PROGRAM AMCI_Motion_Sample
VAR
	
FB_relative_move_1: relative_move_dut; 
b_relative_move_1_en: BOOL;
b_relative_move_1_er: BOOL; 

FB_absolute_move_1: absolute_move_dut; 
b_absolute_move_1_en: BOOL;
b_absolute_move_1_er: BOOL; 

FB_jog_CW_1: jog_cw_dut; 
b_jog_cw_1_en: BOOL;
b_jog_cw_1_er: BOOL; 

FB_jog_CCW_1: jog_ccw_dut; 
b_jog_ccw_1_en: BOOL;
b_jog_ccw_1_er: BOOL; 

FB_home_cw_1: home_cw_dut; 
b_home_cw_1_en: BOOL;
b_home_cw_1_er: BOOL; 

FB_reset_errors_1: reset_errors_dut;  

FB_Preset_1: preset_dut;  
b_preset_1_en: BOOL;
b_preset_1_er: BOOL; 

FB_hold_1: hold_dut;  
b_hold_1_en: BOOL;
b_hold_1_er: BOOL; 

b_comment_coil_1: bool; 

END_VAR
VAR // added by the converter: edge detectors and wires of the graphical bodies
    _w1, _w2, _w3, _w4, _w5, _w6, _w7 : BOOL;
END_VAR

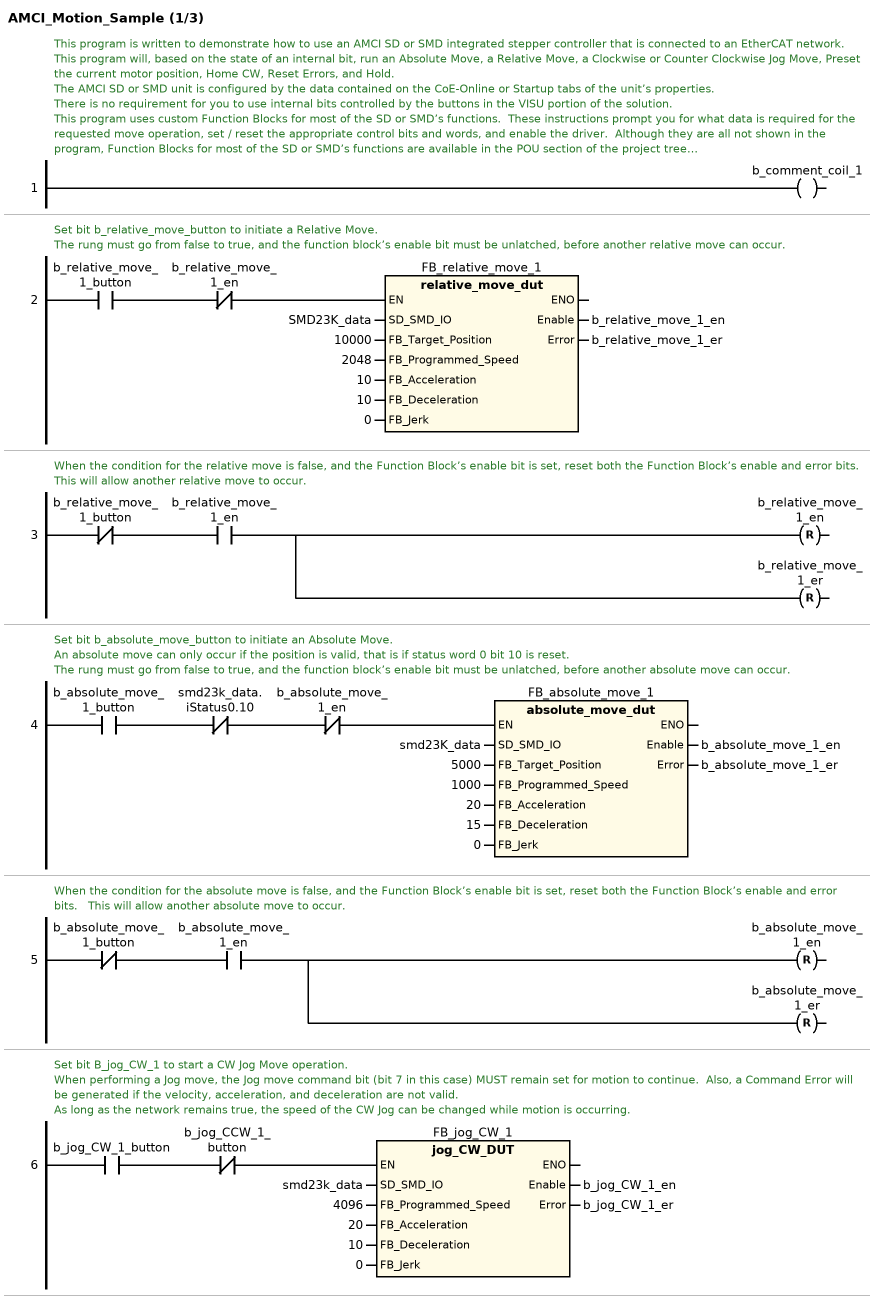
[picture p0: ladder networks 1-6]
// NETWORK 1
// This program is written to demonstrate how to use an AMCI SD or SMD integrated stepper controller that is connected to an EtherCAT network.  This program will, based on the state of an internal bit, run an Absolute Move, a Relative Move, a Clockwise or Counter Clockwise Jog Move, Preset the current motor position, Home CW, Reset Errors, and Hold.
//
// The AMCI SD or SMD unit is configured by the data contained on the CoE-Online or Startup tabs of the unit’s properties.
//
// There is no requirement for you to use internal bits controlled by the buttons in the VISU portion of the solution.
//
// This program uses custom Function Blocks for most of the SD or SMD’s functions.  These instructions prompt you for what data is required for the requested move operation, set / reset the appropriate control bits and words, and enable the driver.  Although they are all not shown in the program, Function Blocks for most of the SD or SMD’s functions are available in the POU section of the project tree.
//
// The custom Function Blocks will only function if a variable with the AMCI_DUT_STEPPER Data Unit Type was linked to the input and output data from the SD or SMD unit.
//
// This program will work correctly only if one button / function is true at a time.
//
// This sample program has a routine containing a Function Block for programming and running Assembled Moves.  Ignore or delete this routine if you are not using this function.
b_comment_coil_1 := TRUE;

// NETWORK 2
// Set bit b_relative_move_button to initiate a Relative Move.
//
// The rung must go from false to true, and the function block’s enable bit must be unlatched, before another relative move can occur.
IF b_relative_move_1_button AND NOT b_relative_move_1_en THEN
    FB_relative_move_1(
        SD_SMD_IO := SMD23K_data,
        FB_Target_Position := 10000,
        FB_Programmed_Speed := 2048,
        FB_Acceleration := 10,
        FB_Deceleration := 10,
        FB_Jerk := 0,
        Enable => b_relative_move_1_en,
        Error => b_relative_move_1_er); // relative_move_dut
END_IF

// NETWORK 3
// When the condition for the relative move is false, and the Function Block’s enable bit is set, reset both the Function Block’s enable and error bits.   This will allow another relative move to occur.
_w1 := NOT b_relative_move_1_button AND b_relative_move_1_en;
b_relative_move_1_en R= _w1;
b_relative_move_1_er R= _w1;

// NETWORK 4
// Set bit b_absolute_move_button to initiate an Absolute Move.
//
// An absolute move can only occur if the position is valid, that is if status word 0 bit 10 is reset.
//
// The rung must go from false to true, and the function block’s enable bit must be unlatched, before another absolute move can occur.
IF b_absolute_move_1_button AND NOT smd23k_data.iStatus0.10 AND NOT b_absolute_move_1_en THEN
    FB_absolute_move_1(
        SD_SMD_IO := smd23K_data,
        FB_Target_Position := 5000,
        FB_Programmed_Speed := 1000,
        FB_Acceleration := 20,
        FB_Deceleration := 15,
        FB_Jerk := 0,
        Enable => b_absolute_move_1_en,
        Error => b_absolute_move_1_er); // absolute_move_dut
END_IF

// NETWORK 5
// When the condition for the absolute move is false, and the Function Block’s enable bit is set, reset both the Function Block’s enable and error bits.   This will allow another absolute move to occur.
_w2 := NOT b_absolute_move_1_button AND b_absolute_move_1_en;
b_absolute_move_1_en R= _w2;
b_absolute_move_1_er R= _w2;

// NETWORK 6
// Set bit B_jog_CW_1 to start a CW Jog Move operation.
//
// When performing a Jog move, the Jog move command bit (bit 7 in this case) MUST remain set for motion to continue.  Also, a Command Error will be generated if the velocity, acceleration, and deceleration are not valid.
//
// As long as the network remains true, the speed of the CW Jog can be changed while motion is occurring.
IF b_jog_CW_1_button AND NOT b_jog_CCW_1_button THEN
    FB_jog_CW_1(
        SD_SMD_IO := smd23k_data,
        FB_Programmed_Speed := 4096,
        FB_Acceleration := 20,
        FB_Deceleration := 10,
        FB_Jerk := 0,
        Enable => b_jog_CW_1_en,
        Error => b_jog_CW_1_er); // jog_CW_DUT
END_IF

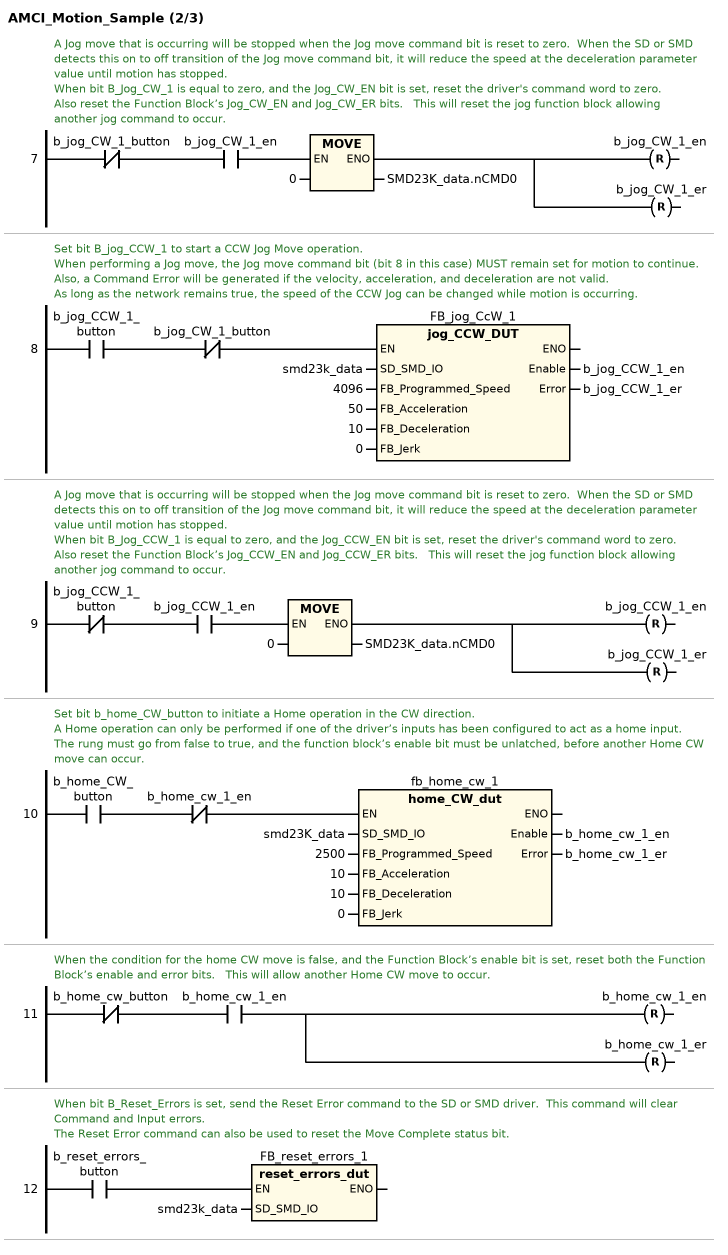
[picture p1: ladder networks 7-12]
// NETWORK 7
// A Jog move that is occurring will be stopped when the Jog move command bit is reset to zero.  When the SD or SMD detects this on to off transition of the Jog move command bit, it will reduce the speed at the deceleration parameter value until motion has stopped.
//
// When bit B_Jog_CW_1 is equal to zero, and the Jog_CW_EN bit is set, reset the driver's command word to zero.
//
// Also reset the Function Block’s Jog_CW_EN and Jog_CW_ER bits.   This will reset the jog function block allowing another jog command to occur.
_w3 := NOT b_jog_CW_1_button AND b_jog_CW_1_en;
IF _w3 THEN SMD23K_data.nCMD0 := 0; END_IF
b_jog_CW_1_en R= _w3;
b_jog_CW_1_er R= _w3;

// NETWORK 8
// Set bit B_jog_CCW_1 to start a CCW Jog Move operation.
//
// When performing a Jog move, the Jog move command bit (bit 8 in this case) MUST remain set for motion to continue.  Also, a Command Error will be generated if the velocity, acceleration, and deceleration are not valid.
//
// As long as the network remains true, the speed of the CCW Jog can be changed while motion is occurring.
IF b_jog_CCW_1_button AND NOT b_jog_CW_1_button THEN
    FB_jog_CcW_1(
        SD_SMD_IO := smd23k_data,
        FB_Programmed_Speed := 4096,
        FB_Acceleration := 50,
        FB_Deceleration := 10,
        FB_Jerk := 0,
        Enable => b_jog_CCW_1_en,
        Error => b_jog_CCW_1_er); // jog_CCW_DUT
END_IF

// NETWORK 9
// A Jog move that is occurring will be stopped when the Jog move command bit is reset to zero.  When the SD or SMD detects this on to off transition of the Jog move command bit, it will reduce the speed at the deceleration parameter value until motion has stopped.
//
// When bit B_Jog_CCW_1 is equal to zero, and the Jog_CCW_EN bit is set, reset the driver's command word to zero.
//
// Also reset the Function Block’s Jog_CCW_EN and Jog_CCW_ER bits.   This will reset the jog function block allowing another jog command to occur.
_w4 := NOT b_jog_CCW_1_button AND b_jog_CCW_1_en;
IF _w4 THEN SMD23K_data.nCMD0 := 0; END_IF
b_jog_CCW_1_en R= _w4;
b_jog_CCW_1_er R= _w4;

// NETWORK 10
// Set bit b_home_CW_button to initiate a Home operation in the CW direction.
//
// A Home operation can only be performed if one of the driver’s inputs has been configured to act as a home input.
//
// The rung must go from false to true, and the function block’s enable bit must be unlatched, before another Home CW move can occur.
IF b_home_CW_button AND NOT b_home_cw_1_en THEN
    fb_home_cw_1(
        SD_SMD_IO := smd23K_data,
        FB_Programmed_Speed := 2500,
        FB_Acceleration := 10,
        FB_Deceleration := 10,
        FB_Jerk := 0,
        Enable => b_home_cw_1_en,
        Error => b_home_cw_1_er); // home_CW_dut
END_IF

// NETWORK 11
// When the condition for the home CW move is false, and the Function Block’s enable bit is set, reset both the Function Block’s enable and error bits.   This will allow another Home CW move to occur.
_w5 := NOT b_home_cw_button AND b_home_cw_1_en;
b_home_cw_1_en R= _w5;
b_home_cw_1_er R= _w5;

// NETWORK 12
// When bit B_Reset_Errors is set, send the Reset Error command to the SD or SMD driver.  This command will clear Command and Input errors.
//
// The Reset Error command can also be used to reset the Move Complete status bit.
IF b_reset_errors_button THEN
    FB_reset_errors_1(SD_SMD_IO := smd23k_data); // reset_errors_dut
END_IF

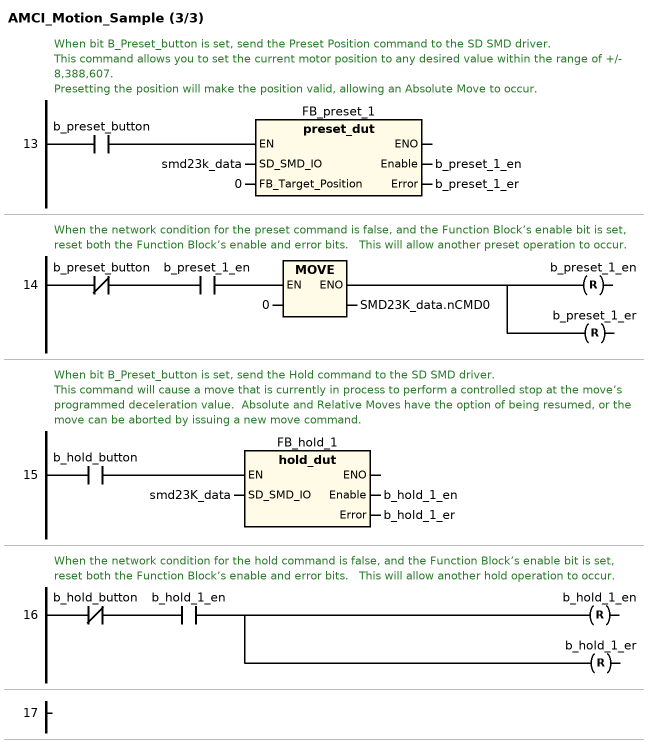
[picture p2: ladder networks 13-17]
// NETWORK 13
// When bit B_Preset_button is set, send the Preset Position command to the SD SMD driver.
//
// This command allows you to set the current motor position to any desired value within the range of +/- 8,388,607.
//
// Presetting the position will make the position valid, allowing an Absolute Move to occur.
IF b_preset_button THEN
    FB_preset_1(
        SD_SMD_IO := smd23k_data,
        FB_Target_Position := 0,
        Enable => b_preset_1_en,
        Error => b_preset_1_er); // preset_dut
END_IF

// NETWORK 14
// When the network condition for the preset command is false, and the Function Block’s enable bit is set, reset both the Function Block’s enable and error bits.   This will allow another preset operation to occur.
_w6 := NOT b_preset_button AND b_preset_1_en;
IF _w6 THEN SMD23K_data.nCMD0 := 0; END_IF
b_preset_1_en R= _w6;
b_preset_1_er R= _w6;

// NETWORK 15
// When bit B_Preset_button is set, send the Hold command to the SD SMD driver.
//
// This command will cause a move that is currently in process to perform a controlled stop at the move’s programmed deceleration value.  Absolute and Relative Moves have the option of being resumed, or the move can be aborted by issuing a new move command.
IF b_hold_button THEN
    FB_hold_1(SD_SMD_IO := smd23K_data, Enable => b_hold_1_en, Error => b_hold_1_er); // hold_dut
END_IF

// NETWORK 16
// When the network condition for the hold command is false, and the Function Block’s enable bit is set, reset both the Function Block’s enable and error bits.   This will allow another hold operation to occur.
_w7 := NOT b_hold_button AND b_hold_1_en;
b_hold_1_en R= _w7;
b_hold_1_er R= _w7;

// NETWORK 17

END_PROGRAM
